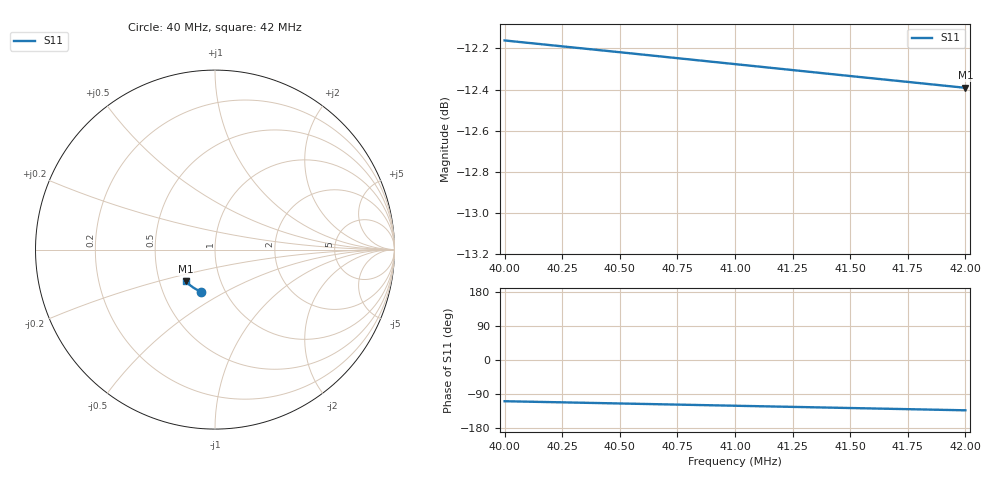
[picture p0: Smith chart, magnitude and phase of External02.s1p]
# Hz S RI R 50
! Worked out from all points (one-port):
!   9 points, 40 MHz to 42 MHz, reference 50 ohm
!   lowest |S11| = -12.4 dB at 42 MHz (marker M1), VSWR 1.63, Z = 34.1 - j12.7 ohm
!   |S11| at or under -10 dB: start of sweep to end of sweep
4e7  -0.0794 -0.2335
4.025e7  -0.091 -0.2283
4.05e7  -0.1025 -0.2225
4.075e7  -0.1135 -0.2161
4.1e7  -0.1243 -0.2092
4.125e7  -0.1346 -0.2017
4.15e7  -0.1445 -0.1937
4.175e7  -0.154 -0.1853
4.2e7  -0.163 -0.1763
